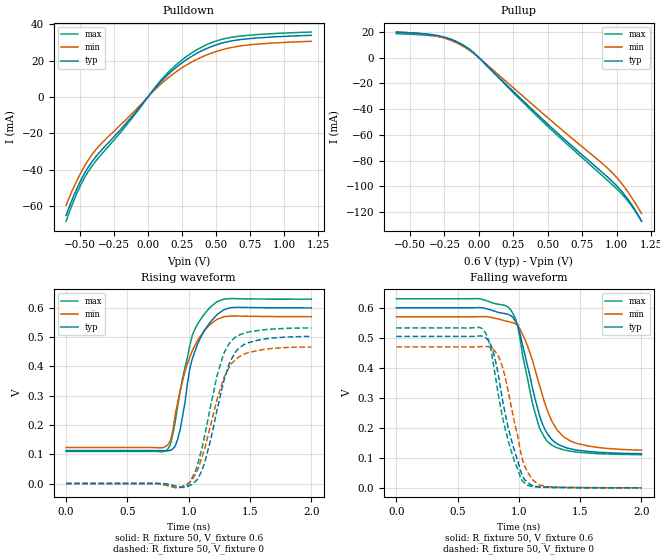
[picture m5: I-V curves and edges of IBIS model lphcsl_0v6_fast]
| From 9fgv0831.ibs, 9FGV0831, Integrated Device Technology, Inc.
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[Model]   lphcsl_0v6_fast
Model_type Output
Polarity Non-Inverting
Enable Active-High
Vmeas = 0.4000V
Cref = 2.0000pF
Rref = 0
Vref = 0.4000V
C_comp 1.1000pF 1.0000pF 1.2000pF
[Temperature Range] 25 75 0
[Voltage Range] 0.6000V 0.5700V 0.6300V
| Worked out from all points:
|   slope of the pulldown table from 0 to 0.09 V, typ, clamps not added: 11.3 ohm
|   slope of the pullup table from 0 to 0.09 V, typ, clamps not added: 9.48 ohm
|   rising waveform, R_fixture 50, V_fixture 0.6: 20-80 % time 160ps typ, 180ps min, 159ps max; typ from 0.113 V to 0.6 V
|   rising waveform, R_fixture 50, V_fixture 0: 20-80 % time 176ps typ, 190ps min, 173ps max; typ from 0 V to 0.503 V
|   falling waveform, R_fixture 50, V_fixture 0.6: 20-80 % time 180ps typ, 217ps min, 161ps max; typ from 0.6 V to 0.114 V
|   falling waveform, R_fixture 50, V_fixture 0: 20-80 % time 163ps typ, 145ps min, 164ps max; typ from 0.504 V to 0 V
[Pulldown]
|Voltage I(typ) I(min) I(max)
-600mV    -65.21mA   -59.64mA   -68.48mA
-540mV    -53.77mA   -49.11mA   -56.45mA
-500mV    -47.15mA   -42.93mA   -49.62mA
-440mV    -38.96mA   -35.03mA   -41.34mA
-380mV    -32.74mA   -28.88mA   -35.09mA
-140mV    -12.81mA   -10.93mA   -13.94mA
100mV     8.769mA    7.433mA    9.577mA
260mV     19.34mA    16.56mA    21mA
420mV     26.34mA    22.82mA    28.41mA
580mV     30.41mA    26.74mA    32.45mA
800mV     32.55mA    29.15mA    34.41mA
1.2V      34.02mA    30.72mA    35.83mA
[Pullup]
|Voltage I(typ) I(min) I(max)
-600mV    19.81mA    19.9mA     18.63mA
-380mV    18.39mA    18.13mA    17.44mA
-260mV    16.25mA    15.47mA    15.78mA
-160mV    12.32mA    11.36mA    12.3mA
-60mV     5.642mA    5.048mA    5.78mA
0V        720.8pA    1.104nA    645pA
480mV     -49.7mA    -44.85mA   -51.38mA
940mV     -93.39mA   -86.48mA   -95.95mA
1V        -99.57mA   -93.12mA   -101.9mA
1.06V     -107mA     -101.1mA   -108.6mA
1.12V     -116mA     -110.5mA   -116.9mA
1.18V     -126.7mA   -121.1mA   -127.1mA
[Ramp]
| variable typ min max
dV/dt_r 0.3017/0.1766n 0.2797/0.1900n 0.3191/0.1728n
dV/dt_f 0.2917/0.1873n 0.2666/0.2169n 0.3116/0.1771n
R_load = 50
[Rising Waveform]
R_fixture= 50
V_fixture= 0.6
V_fixture_min= 0.57
V_fixture_max= 0.63
|time V(typ) V(min) V(max)
0s        112.6mV    123mV      109.7mV
810ps     111.8mV    125.8mV    111.1mV
850ps     113.2mV    146mV      132.5mV
910ps     151.4mV    276.4mV    264.1mV
970ps     277.8mV    382.9mV    397.8mV
1.01ns    394.9mV    432.9mV    473.6mV
1.03ns    426.8mV    454.8mV    507.4mV
1.17ns    548.2mV    541.3mV    600.3mV
1.33ns    599.8mV    571.9mV    631.7mV
2ns       600.1mV    570.3mV    630.1mV
[Rising Waveform]
R_fixture= 50
V_fixture= 0
V_fixture_min= 0
V_fixture_max= 0
|time V(typ) V(min) V(max)
0s        0V         0V         0V
990ps     -10.88mV   -1.163mV   -4.753mV
1.07ns    13.16mV    43.5mV     60.52mV
1.13ns    70.91mV    118.7mV    162.5mV
1.23ns    248.4mV    285.1mV    366.2mV
1.29ns    356mV      364.6mV    448.2mV
1.35ns    426.1mV    410.1mV    489.3mV
1.39ns    454.8mV    426.7mV    503.1mV
1.49ns    482mV      447.8mV    518.2mV
2ns       502.9mV    466.2mV    531.9mV
[Falling Waveform]
R_fixture= 50
V_fixture= 0.6
V_fixture_min= 0.57
V_fixture_max= 0.63
|time V(typ) V(min) V(max)
0s        600mV      570mV      630mV
670ps     600.4mV    570.1mV    630.3mV
910ps     578.4mV    554.2mV    603mV
990ps     544mV      540.9mV    539.4mV
1.05ns    441.8mV    494.3mV    403.9mV
1.15ns    268.4mV    367.7mV    224.1mV
1.23ns    181.9mV    260.5mV    155.5mV
1.31ns    147.6mV    193.6mV    133.8mV
1.43ns    129.2mV    154.7mV    121.6mV
2ns       113.8mV    125.6mV    110.6mV
[Falling Waveform]
R_fixture= 50
V_fixture= 0
V_fixture_min= 0
V_fixture_max= 0
|time V(typ) V(min) V(max)
0s        504.4mV    469.5mV    532.8mV
710ps     504.7mV    470.8mV    527mV
750ps     491.6mV    470.5mV    495.3mV
790ps     455.1mV    462mV      418.3mV
850ps     333.2mV    423.2mV    270.3mV
950ps     142.8mV    246.4mV    106.9mV
1.03ns    38.06mV    92.3mV     21.97mV
1.07ns    19.06mV    53.05mV    8.341mV
1.23ns    2.108mV    4.368mV    1.591mV
2ns       93.89uV    172.9uV    66.57uV
